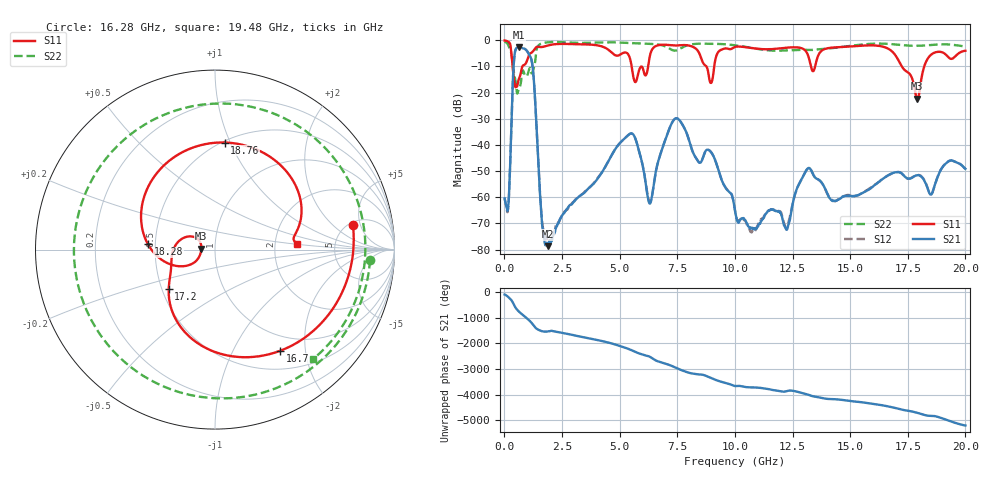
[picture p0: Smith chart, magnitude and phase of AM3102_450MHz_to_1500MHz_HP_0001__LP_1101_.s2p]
!Agilent Technologies,E8364B,MY43040894,A.07.50.67
!Agilent E8364B: A.07.50.67
!Date: Thursday, January 11, 2018 05:22:43
!Correction: S11(Full 2 Port(1,2))
!S21(Full 2 Port(1,2))
!S12(Full 2 Port(1,2))
!S22(Full 2 Port(1,2))
!S2P File: Measurements: S11, S21, S12, S22:
# Hz S  dB  R 50
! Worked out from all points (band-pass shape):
!   1601 points, 10 MHz to 20 GHz, reference 50 ohm
!   highest |S21| = -2.67 dB at 622.2 MHz (marker M1); lowest = -78.7 dB at 1.897 GHz (marker M2)
!   |S21| within 3 dB of the highest: 440.1 MHz to 1.09 GHz (649.8 MHz wide, 84.9 % of centre)
!   lowest |S11| = -22.4 dB at 17.91 GHz (marker M3), VSWR 1.16, Z = 42.9 + j0.402 ohm
!   |S11| at or under -10 dB: 357.5 MHz to 780.4 MHz (422.9 MHz wide, 74.3 % of centre); 5.522 GHz to 6.238 GHz (715.2 MHz wide, 12.2 % of centre); 17.24 GHz to 18.21 GHz (971.1 MHz wide, 5.48 % of centre)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
!   |S22| runs from -20.4 to -0.5 dB; largest |S21 - S12| = 0.0019
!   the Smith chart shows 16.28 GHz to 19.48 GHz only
!   S11 on the Smith chart (normalised r, x): 16.28 GHz: 5.42, +3.77; 16.7 GHz: 0.76, -1.56; 17.2 GHz: 0.54, -0.27; 18.28 GHz: 0.46, +0.03; 18.76 GHz: 0.51, +0.95; 19.48 GHz: 2.67, +0.20
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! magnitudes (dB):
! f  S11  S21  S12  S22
! 10 MHz  -0.1  -60.4  -60.1  -0.5
! 622.2 MHz  -15.0  -2.7  -2.7  -18.8
! 1.197 GHz  -4.6  -8.4  -8.4  -12.6
! 1.622 GHz  -2.6  -69.0  -67.6  -1.2
! 1.897 GHz  -2.0  -78.7  -76.5  -0.8
! 3.346 GHz  -1.5  -58.9  -59.1  -1.0
! 5.445 GHz  -6.8  -35.7  -35.7  -1.0
! 6.294 GHz  -6.7  -62.3  -61.9  -1.3
! 6.682 GHz  -1.9  -46.0  -46.0  -1.6
! 7.531 GHz  -1.9  -30.0  -30.0  -3.6
! 10.01 GHz  -2.5  -65.0  -65.2  -1.9
! 12.24 GHz  -2.8  -72.4  -71.4  -3.9
! 13.34 GHz  -11.3  -50.2  -50.2  -3.7
! 16.28 GHz  -2.2  -54.0  -53.9  -1.3
! 16.68 GHz  -3.3  -51.4  -51.5  -1.4
! 16.7 GHz  -3.5  -51.3  -51.4  -1.4
! 17.2 GHz  -9.4  -50.7  -50.6  -1.8
! 17.91 GHz  -22.4  -51.6  -51.5  -2.1
! 18.28 GHz  -8.5  -54.6  -54.4  -1.9
! 18.76 GHz  -4.4  -53.0  -52.9  -1.6
! 19.48 GHz  -6.8  -46.1  -46.1  -1.7
! 20 GHz  -4.0  -49.1  -49.1  -2.3
